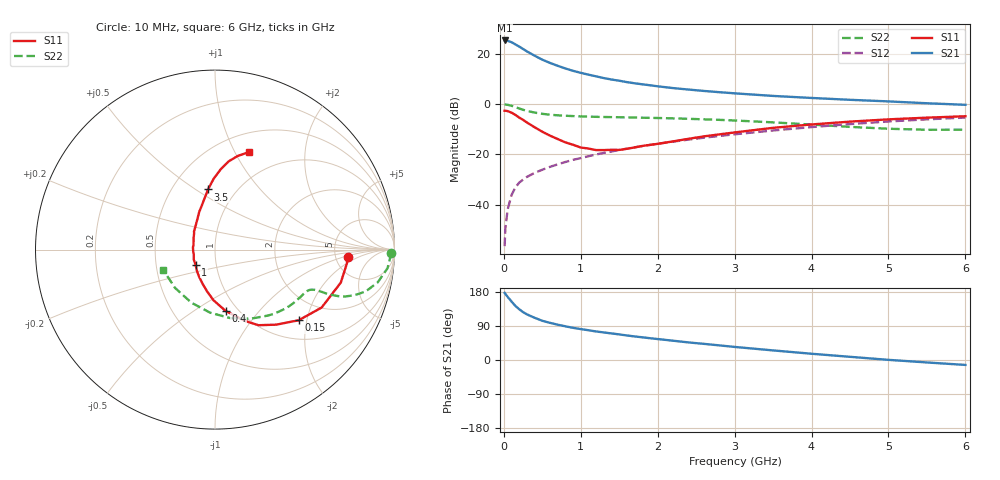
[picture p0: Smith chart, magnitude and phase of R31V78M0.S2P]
! SIEMENS Small Signal Semiconductors
! BFR181
! Si NPN RF Bipolar Junction Transistor in SOT23
! VCE = 1.75 V  IC = 8 mA
! Common Emitter S-Parameters:  May  1996
# GHz  S  MA  R  50
!  f  S11  S21  S12  S22
! GHz  MAG  ANG  MAG  ANG  MAG  ANG  MAG  ANG
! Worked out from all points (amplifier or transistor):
!   36 points, 10 MHz to 6 GHz, reference 50 ohm
!   highest |S21| = 25.3 dB at 10 MHz (marker M1)
!   |S21| within 3 dB of that: start of sweep to 229.7 MHz
!   unconditionally stable (mu >= 1): 763.7 MHz to 2.779 GHz
!   at 250 MHz: K = 0.57, MSG = 26.0 dB, |S12| = -30.0 dB
!   at 1.4 GHz: K = 1.08, MAG = 12.5 dB, |S12| = -18.8 dB
!   at 6 GHz: K = 0.86, MSG = 2.5 dB, |S12| = -5.3 dB
!   S11 on the Smith chart (normalised r, x): 10 MHz: 6.45, -1.21; 150 MHz: 1.43, -1.79; 400 MHz: 0.88, -0.68; 1 GHz: 0.79, -0.14; 3.5 GHz: 0.74, +0.56; 6 GHz: 0.70, +1.14
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0.01  0.7396 -3.3  18.4 177.2  0.0015 87.2  0.9822 -1.1
0.02  0.7391 -5.9  18.13 174.3  0.0034 86.2  0.9777 -2.5
0.05  0.7246 -14.7  18.03 166.5  0.0081 81.5  0.9666 -6.2
0.1  0.6763 -28.5  16.98 154.2  0.0156 77.6  0.9247 -11.4
0.15  0.61 -40.2  15.36 142.8  0.0221 71.7  0.8717 -15.5
0.2  0.5397 -50.8  13.91 133.9  0.0275 69.1  0.818 -18.1
0.25  0.4859 -60.1  12.45 126.3  0.0315 67.0  0.771 -19.8
0.3  0.4305 -67.3  11.15 120.4  0.0357 66.1  0.7334 -20.7
0.4  0.3466 -80.2  9.161 111.4  0.0429 65.5  0.6781 -21.5
0.5  0.282 -91.8  7.632 103.5  0.0496 65.9  0.64 -21.6
0.6  0.2358 -101.0  6.581 98.0  0.0566 66.6  0.6144 -21.8
0.7  0.2021 -110.1  5.768 93.2  0.0634 66.9  0.5983 -22.0
0.8  0.1733 -121.3  5.104 88.9  0.0707 67.0  0.5865 -22.4
1  0.137 -142.3  4.177 81.6  0.0845 68.1  0.5692 -23.4
1.1  0.1309 -154.5  3.844 78.5  0.092 68.4  0.5635 -24.1
1.3  0.1218 -174.6  3.288 72.7  0.1073 68.2  0.5539 -25.9
1.6  0.1292 157.2  2.734 64.7  0.1302 67.6  0.544 -29.1
2.2  0.1815 124.8  2.08 50.9  0.1796 64.8  0.5198 -37.3
3.5  0.3374 96.6  1.453 25.3  0.2989 54.6  0.4334 -62.7
4.5  0.4482 86.0  1.216 8.4  0.4008 43.4  0.3523 -94.5
5.5  0.5373 76.3  1.039 -6.5  0.4975 30.0  0.3085 -136.3
6  0.5736 71.0  0.967 -13.0  0.5404 22.7  0.3099 -158.7
